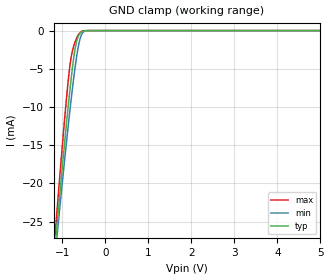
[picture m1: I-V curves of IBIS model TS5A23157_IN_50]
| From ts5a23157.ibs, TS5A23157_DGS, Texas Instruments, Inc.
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[Model]   TS5A23157_IN_50
Model_type  Input
Vinl=1.65
Vinh=3.15
| variable   typ   min   max
C_comp   2.45pF   1.90pF   3.43pF
[Temperature Range]   40   100   -40
| Ambient temperature   25   85   -40
[Voltage range]   5   4.5   5.5
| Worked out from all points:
|   GND clamp passes 1 mA (typ) near -0.64 V on its own axis
[GND Clamp]
| TS5A23157_IN_50
|   Voltage   I(typ)   I(min)   I(max)
-5V       -302.2mA   -280.5mA   -327.4mA
-1.155V   -27.79mA   -28.96mA   -26.1mA
-1.12V    -25.56mA   -26.93mA   -23.62mA
-1.085V   -23.36mA   -24.92mA   -21.17mA
-925mV    -13.66mA   -15.99mA   -10.47mA
-815mV    -7.538mA   -10.24mA   -4.411mA
-760mV    -4.83mA    -7.556mA   -2.626mA
-680mV    -1.807mA   -4.063mA   -1.206mA
-605mV    -517.4uA   -1.575mA   -393.5uA
-545mV    -167.7uA   -480.8uA   -102.2uA
-400mV    -4.863uA   -10.82uA   -937.9nA
5V        123.2pA    299.2pA    65.41pA
